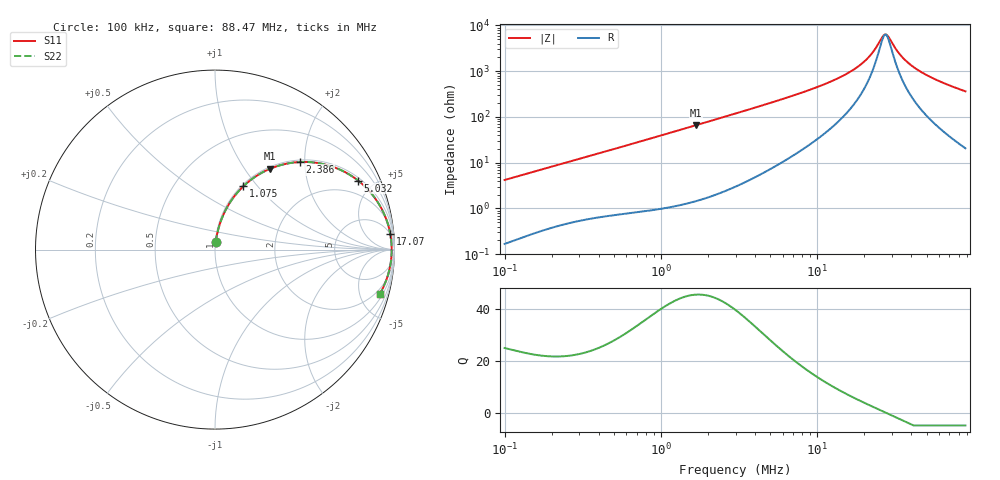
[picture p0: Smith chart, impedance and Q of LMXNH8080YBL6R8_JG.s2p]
! LMXNH8080YBL6R8_JG  S-PARAMETER MODEL  ( General Type )
! Model Generated by TAIYO YUDEN Corporation (https://www.yuden.co.jp/en/)
! Version 1.0
! TAIYO YUDEN Control No. 191025NI43SB-FBB
! Copyright(c) 2019 TAIYO YUDEN CO.,LTD. All Rights Reserved.
! Product Description (link to TY-COMPAS)
! https://ds.yuden.co.jp/TYCOMPAS/or/detail?pn=LMXNH8080YBL6R8NJG&u=M
! Products Name : Inductors
! Characteristics :
!  Inductance : 6.8 uH , SRF(min) : 24 MHz , DC Resistance(max) : 0.0325 Ohm
!  Rated Current : Saturation :4400 mA , Temp Rise : 3700 mA (40 degC)
!  Case Size : 8.0 x 8.0 / 0.315 x 0.315 [mm/inch] , Thickness : 4.2 / 0.165 [mm/inch]
!  (Conditions: Temperature = 25 degC , DC Bias Current/Voltage = 0A / 0V)
! External Node Assignments :
!  1  o---GGG---o  2
! GND o---------o GND
! Frequency Range : 0.1MHz  -  88.465963MHz  [ 402 STEP ]
# MHz S RI R 50
! Freq[MHz].  S11 Real  S11 Imag  S21 Real  S21 Imag  S12 Real  S12 Imag  S22 Real  S22 Imag
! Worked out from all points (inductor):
!   401 points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, 100 kHz to 88.47 MHz, reference 50 ohm
!   read as one part in series: L = 6.63 uH near 103.5 kHz
!   highest Q = 45.6 at 1.671 MHz (marker M1), where L = 6.27 uH
!   self-resonance near 26.98 MHz
!   S11 on the Smith chart (normalised r, x): 100 kHz: 1.00, +0.08; 1.075 MHz: 1.02, +0.85; 2.386 MHz: 1.04, +1.89; 5.032 MHz: 1.15, +4.08; 17.07 MHz: 5, +21; 88.47 MHz: 1.41, -7.26
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0.1  0.00342 0.0417  0.9966 -0.0417  0.9966 -0.0417  0.00342 0.0417
0.311591  0.0207 0.1223  0.9793 -0.1223  0.9793 -0.1223  0.0207 0.1223
0.593648  0.0589 0.2196  0.9411 -0.2196  0.9411 -0.2196  0.0589 0.2196
0.97089  0.1339 0.3282  0.8661 -0.3282  0.8661 -0.3282  0.1339 0.3282
1.074909  0.158 0.3528  0.842 -0.3528  0.842 -0.3528  0.158 0.3528
1.670753  0.3062 0.4501  0.6938 -0.4501  0.6938 -0.4501  0.3062 0.4501
2.385711  0.4713 0.4878  0.5287 -0.4878  0.5287 -0.4878  0.4713 0.4878
2.974323  0.5801 0.4811  0.4199 -0.4811  0.4199 -0.4811  0.5801 0.4811
5.032262  0.798 0.3839  0.202 -0.3839  0.202 -0.3839  0.798 0.3839
9.267725  0.9306 0.223  0.0694 -0.223  0.0694 -0.223  0.9306 0.223
13.23363  0.9641 0.1398  0.0359 -0.1398  0.0359 -0.1398  0.9641 0.1398
17.06801  0.9766 0.0874  0.0234 -0.0874  0.0234 -0.0874  0.9766 0.0874
19.54873  0.9807 0.0612  0.0193 -0.0612  0.0193 -0.0612  0.9807 0.0612
21.64313  0.9827 0.0422  0.0173 -0.0422  0.0173 -0.0422  0.9827 0.0422
26.52916  0.9845 0.00499  0.0155 -0.00499  0.0155 -0.00499  0.9845 0.00499
27.44463  0.9846 -0.00116  0.0154 0.00116  0.0154 0.00116  0.9846 -0.00116
28.8774  0.9844 -0.0104  0.0156 0.0104  0.0156 0.0104  0.9844 -0.0104
31.97126  0.9837 -0.0289  0.0163 0.0289  0.0163 0.0289  0.9837 -0.0289
34.21587  0.9828 -0.0414  0.0172 0.0414  0.0172 0.0414  0.9828 -0.0414
41.94023  0.978 -0.08  0.022 0.08  0.022 0.08  0.978 -0.08
57.88989  0.9623 -0.1464  0.0377 0.1464  0.0377 0.1464  0.9623 -0.1464
88.46596  0.9175 -0.2481  0.0825 0.2481  0.0825 0.2481  0.9175 -0.2481
